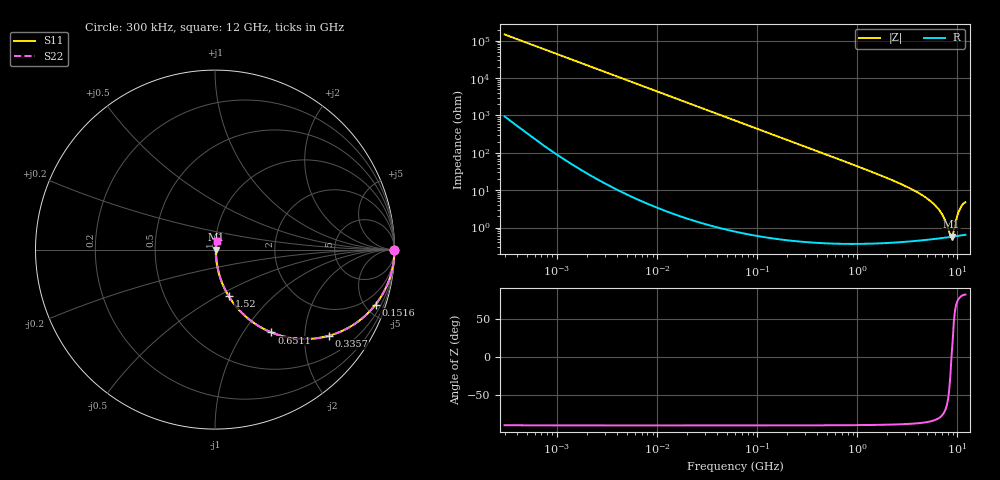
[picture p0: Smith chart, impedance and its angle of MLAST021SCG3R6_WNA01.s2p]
! MLAST021SCG3R6_WNA01  S-PARAMETER MODEL  ( General Type )
! Model Generated by TAIYO YUDEN Corporation (http://www.ty-top.com)
! Version 1.0
! TAIYO YUDEN Control No. 220901
! Copyright(c) 2022 TAIYO YUDEN CO.,LTD. All Rights Reserved.
! Product Description (link to TY-COMPAS)
! https://ds.yuden.co.jp/TYCOMPAS/or/detail?pn=MLAST021SCG3R6BWNA01&u=M
! Products Name : Multilayer Ceramic Capacitors
! Characteristics :
!  Capacitance : 3.6 pF , Rated Voltage : 25V , TCC : CG / C0G
!  Case Size : 0.25 x 0.125 / 0.0098 x 0.0049 [mm/inch] , Thickness : 0.125 / 0.0049 [mm/inch]
!  (Conditions: Temperature = 25 degC , DC Bias Current/Voltage = 0A / 0V)
! External Node Assignments :
!  1  o---| |---o  2
! GND o---------o GND
! Frequency Range : 0.3MHz  -  12000MHz  [ 401 STEP ]
# MHz S RI R 50
! Freq[MHz].  S11 Real  S11 Imag  S21 Real  S21 Imag  S12 Real  S12 Imag  S22 Real  S22 Imag
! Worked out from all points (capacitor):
!   401 points, 300 kHz to 12 GHz, reference 50 ohm
!   read as one part in series: C = 3.6 pF near 316.3 kHz
!   lowest |Z| = 565 mohm at 8.732 GHz (marker M1)
!   series resonance near 8.714 GHz, so ESL is about 93 pH
!   S11 on the Smith chart (normalised r, x): 300 kHz: open; 151.6 MHz: 1.01, -5.83; 335.7 MHz: 1.01, -2.63; 651.1 MHz: 1.01, -1.35; 1.52 GHz: 1.01, -0.56; 12 GHz: 1.01, +0.09
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0.3  1 -0.000679  4.79e-06 0.000679  4.79e-06 0.000679  1 -0.000679
1.769972  1 -0.004  2.15e-05 0.004  2.15e-05 0.004  1 -0.004
10.44266  0.9994 -0.0236  0.000576 0.0236  0.000576 0.0236  0.9994 -0.0236
60  0.9818 -0.1332  0.0182 0.1332  0.0182 0.1332  0.9818 -0.1332
151.6462  0.8943 -0.3067  0.1057 0.3067  0.1057 0.3067  0.8943 -0.3067
335.7268  0.6332 -0.4804  0.3668 0.4804  0.3668 0.4804  0.6332 -0.4804
353.9943  0.6082 -0.4866  0.3918 0.4866  0.3918 0.4866  0.6082 -0.4866
651.0506  0.3141 -0.4614  0.6859 0.4614  0.6859 0.4614  0.3141 -0.4614
994.7115  0.1634 -0.3656  0.8366 0.3656  0.8366 0.3656  0.1634 -0.3656
1519.776  0.0766 -0.2595  0.9234 0.2595  0.9234 0.2595  0.0766 -0.2595
2088.533  0.0417 -0.1904  0.9583 0.1904  0.9583 0.1904  0.0417 -0.1904
3841.137  0.0128 -0.0911  0.9872 0.0911  0.9872 0.0911  0.0128 -0.0911
5565.855  0.007 -0.0464  0.993 0.0464  0.993 0.0464  0.007 -0.0464
6879.757  0.00574 -0.0239  0.9943 0.0239  0.9943 0.0239  0.00574 -0.0239
7448.838  0.00556 -0.0158  0.9944 0.0158  0.9944 0.0158  0.00556 -0.0158
8281.503  0.00554 -0.00507  0.9945 0.00507  0.9945 0.00507  0.00554 -0.00507
8732.115  0.00562 0.000202  0.9944 -0.000202  0.9944 -0.000202  0.00562 0.000202
9207.246  0.00577 0.00621  0.9942 -0.00621  0.9942 -0.00621  0.00577 0.00621
9968.853  0.00629 0.0196  0.9937 -0.0196  0.9937 -0.0196  0.00629 0.0196
10511.28  0.00684 0.0285  0.9932 -0.0285  0.9932 -0.0285  0.00684 0.0285
11380.75  0.00797 0.0417  0.992 -0.0417  0.992 -0.0417  0.00797 0.0417
12000  0.00851 0.0464  0.9915 -0.0464  0.9915 -0.0464  0.00851 0.0464
